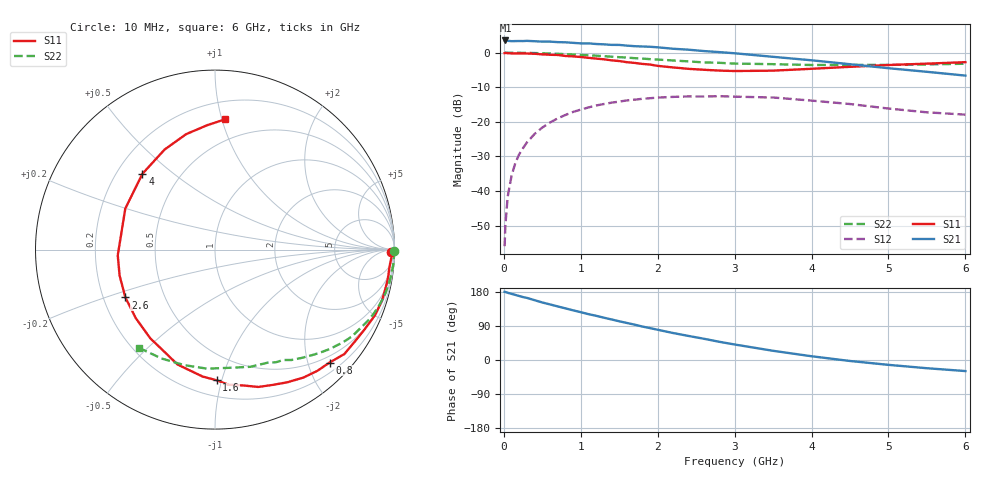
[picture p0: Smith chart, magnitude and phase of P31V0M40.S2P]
! SIEMENS Small Signal Semiconductors
! BFP181
! Si NPN RF Bipolar Junction Transistor in SOT143
! VCE = 1 V  IC = 0.4 mA
! Common Emitter S-Parameters:  March  1996
# GHz  S  MA  R  50
!  f  S11  S21  S12  S22
! GHz  MAG  ANG  MAG  ANG  MAG  ANG  MAG  ANG
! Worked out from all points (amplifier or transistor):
!   36 points, 10 MHz to 6 GHz, reference 50 ohm
!   highest |S21| = 3.5 dB at 20 MHz (marker M1)
!   |S21| within 3 dB of that: start of sweep to 2.568 GHz
!   unconditionally stable (mu >= 1): 3.718 GHz to end of sweep
!   at 250 MHz: K = 0.08, MSG = 15.5 dB, |S12| = -27.6 dB
!   at 1.4 GHz: K = 0.46, MSG = 8.4 dB, |S12| = -14.5 dB
!   at 6 GHz: K = 1.60, MAG = 1.1 dB, |S12| = -17.9 dB
!   S11 on the Smith chart (normalised r, x): 10 MHz: 77, -53; 800 MHz: 0.37, -2.39; 1.6 GHz: 0.31, -0.96; 2.6 GHz: 0.29, -0.23; 4 GHz: 0.31, +0.39; 6 GHz: 0.33, +1.03
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0.01  0.9825 -0.7  1.483 179.8  0.0016 84.4  0.9997 -0.3
0.02  0.9904 -1.2  1.501 179.6  0.0032 89.4  0.9997 -0.6
0.05  0.9831 -2.7  1.483 177.4  0.0083 91.2  0.9991 -1.4
0.1  0.9767 -5.8  1.466 174.5  0.0166 86.2  0.9973 -2.8
0.15  0.9767 -8.4  1.47 171.8  0.0256 83.1  0.9974 -4.2
0.2  0.9754 -11.1  1.473 168.8  0.0341 81.8  0.9955 -5.6
0.3  0.9727 -16.9  1.481 163.9  0.0505 78.0  0.992 -8.5
0.4  0.9639 -22.2  1.463 157.8  0.0669 73.9  0.9874 -11.3
0.6  0.932 -33.5  1.444 146.7  0.0979 65.5  0.9722 -16.9
0.8  0.8963 -44.6  1.412 136.3  0.1258 57.7  0.9525 -22.2
1.1  0.8419 -61.4  1.363 121.0  0.1616 46.5  0.9154 -29.5
1.3  0.8024 -72.5  1.319 111.7  0.1811 39.1  0.8901 -34.4
1.6  0.7279 -89.3  1.264 97.7  0.2041 30.0  0.8496 -40.5
1.9  0.6734 -108.1  1.217 84.2  0.2198 20.8  0.806 -46.4
2.2  0.6117 -126.1  1.139 71.2  0.2296 12.8  0.7705 -51.7
2.6  0.5661 -151.9  1.055 56.1  0.2325 3.2  0.723 -58.3
3  0.5427 -176.6  0.98 40.9  0.2314 -6.4  0.695 -65.0
3.5  0.5496 155.4  0.871 24.3  0.2249 -15.8  0.6821 -73.2
4  0.5848 133.7  0.776 9.9  0.2029 -23.7  0.6635 -83.0
4.5  0.6243 116.7  0.681 -2.6  0.1811 -30.1  0.6648 -93.8
5.5  0.694 93.7  0.529 -21.7  0.1374 -30.4  0.6759 -116.2
6  0.7293 85.4  0.466 -29.2  0.1273 -26.5  0.6919 -127.7
